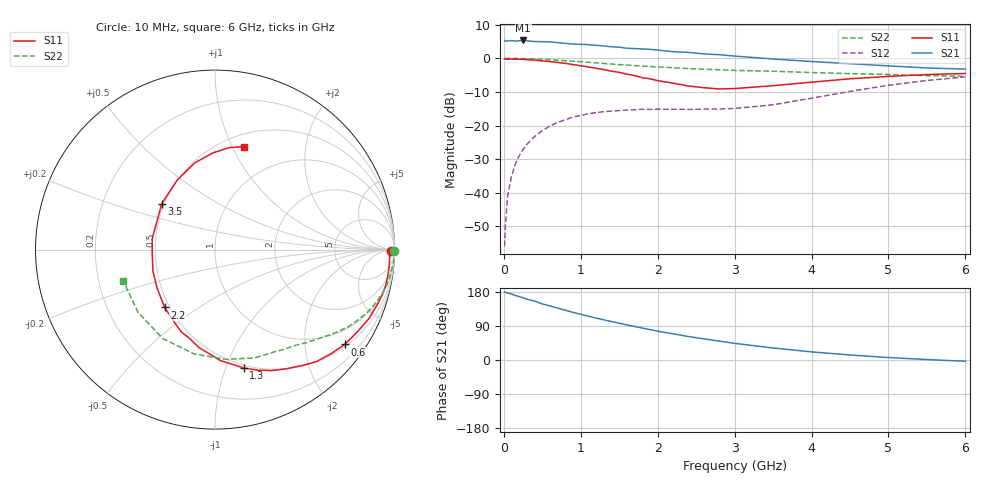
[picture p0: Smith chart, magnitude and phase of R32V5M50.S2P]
! SIEMENS Small Signal Semiconductors
! BFR181
! Si NPN RF Bipolar Junction Transistor in SOT23
! VCE = 2.5 V  IC = 0.5 mA
! Common Emitter S-Parameters:  May  1996
# GHz  S  MA  R  50
!  f  S11  S21  S12  S22
! GHz  MAG  ANG  MAG  ANG  MAG  ANG  MAG  ANG
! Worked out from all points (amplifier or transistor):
!   36 points, 10 MHz to 6 GHz, reference 50 ohm
!   highest |S21| = 5.3 dB at 250 MHz (marker M1)
!   |S21| within 3 dB of that: start of sweep to 2.054 GHz
!   unconditionally stable (mu >= 1): 2.353 GHz to 3.989 GHz
!   at 250 MHz: K = 0.13, MSG = 16.2 dB, |S12| = -27.2 dB
!   at 1.4 GHz: K = 0.61, MSG = 9.6 dB, |S12| = -15.7 dB
!   at 6 GHz: K = 0.92, MSG = 1.2 dB, |S12| = -5.5 dB
!   S11 on the Smith chart (normalised r, x): 10 MHz: open; 600 MHz: 0.56, -2.97; 1.3 GHz: 0.47, -1.16; 2.2 GHz: 0.47, -0.37; 3.5 GHz: 0.48, +0.29; 6 GHz: 0.62, +1.11
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0.01  0.9829 -0.6  1.837 179.7  0.0016 96.7  0.9996 -0.4
0.02  0.9725 -1.0  1.81 178.6  0.0032 89.0  0.9936 -0.6
0.05  0.9744 -3.1  1.812 177.1  0.0091 86.4  0.9983 -1.4
0.1  0.9752 -6.0  1.836 174.2  0.0176 86.5  0.9992 -2.8
0.15  0.9738 -9.0  1.807 170.1  0.0268 83.6  0.9953 -4.5
0.25  0.9651 -15.1  1.846 164.0  0.0438 79.1  0.9898 -7.2
0.4  0.94 -24.1  1.781 155.4  0.0686 73.3  0.9779 -11.4
0.5  0.9155 -30.2  1.769 148.1  0.0839 69.3  0.9667 -14.1
0.6  0.8951 -36.2  1.759 142.6  0.0982 65.1  0.9523 -16.8
0.8  0.842 -47.8  1.67 131.3  0.1224 58.0  0.9216 -21.7
1.1  0.7438 -65.0  1.598 115.6  0.1493 48.8  0.8725 -28.2
1.3  0.6795 -76.3  1.53 106.0  0.1608 43.8  0.8386 -32.0
1.8  0.5153 -105.8  1.381 84.2  0.1746 35.8  0.768 -39.7
2  0.4656 -118.7  1.326 76.0  0.1755 34.2  0.7455 -42.7
2.2  0.4274 -131.1  1.256 69.1  0.1745 33.3  0.725 -45.8
2.4  0.3876 -146.2  1.225 61.9  0.1735 34.2  0.7035 -48.7
2.8  0.3502 -176.2  1.133 49.9  0.1762 37.3  0.677 -55.2
3.5  0.3919 139.1  0.977 31.7  0.2037 46.6  0.6427 -70.0
4.5  0.4963 103.1  0.833 13.3  0.3227 49.6  0.5928 -101.4
5  0.5386 91.3  0.772 6.5  0.3971 44.5  0.5744 -120.6
5.5  0.5739 82.1  0.719 1.2  0.4682 36.8  0.553 -140.8
6  0.5951 74.5  0.692 -3.3  0.5299 28.1  0.5406 -161.1
